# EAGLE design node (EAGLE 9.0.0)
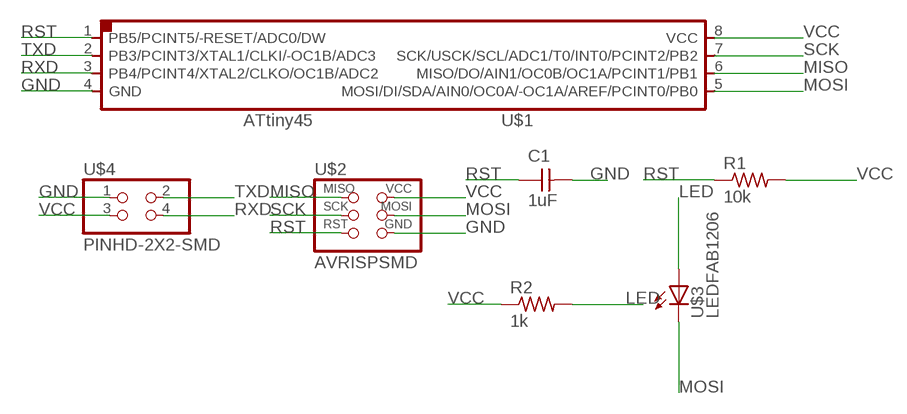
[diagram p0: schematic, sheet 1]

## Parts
C1  1uF  CAP-UNPOLARIZEDFAB  [C1206FAB]
R1  10k  RES-US1206FAB  [R1206FAB]
R2  1k  RES-US1206FAB  [R1206FAB]
U$1  ATTINY45SI  [SOIC8]
U$2  AVRISPSMD  [2X03SMD]
U$3  LEDFAB1206  [LED1206FAB]
U$4  PINHD-2X2-SMD  [2X02SMD]

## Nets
GND: C1.2 U$1.4(GND) U$2.6(GND) U$4.1
LED: R2.2 U$3.1(A)
MISO: U$1.6(MISO/DO/AIN1/OC0B/OC1A/PCINT1/PB1) U$2.1(MISO)
MOSI: U$1.5(MOSI/DI/SDA/AIN0/OC0A/-OC1A/AREF/PCINT0/PB0) U$2.4(MOSI) U$3.2(C)
RST: C1.1 R1.1 U$1.1(PB5/PCINT5/-RESET/ADC0/DW) U$2.5(RST)
RXD: U$1.3(PB4/PCINT4/XTAL2/CLKO/OC1B/ADC2) U$4.4
SCK: U$1.7(SCK/USCK/SCL/ADC1/T0/INT0/PCINT2/PB2) U$2.3(SCK)
TXD: U$1.2(PB3/PCINT3/XTAL1/CLKI/-OC1B/ADC3) U$4.2
VCC: R1.2 R2.1 U$1.8(VCC) U$2.2(VCC) U$4.3

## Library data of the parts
C1 = fab:CAP-UNPOLARIZED
R1 R2 = fab:RES-US: Resistor (US Symbol)
U$1 = fab:ATTINY45
U$2 = fab:AVRISP
U$3 = fab:LED: LED
U$4 = fab:PINHD-2X2-SMD

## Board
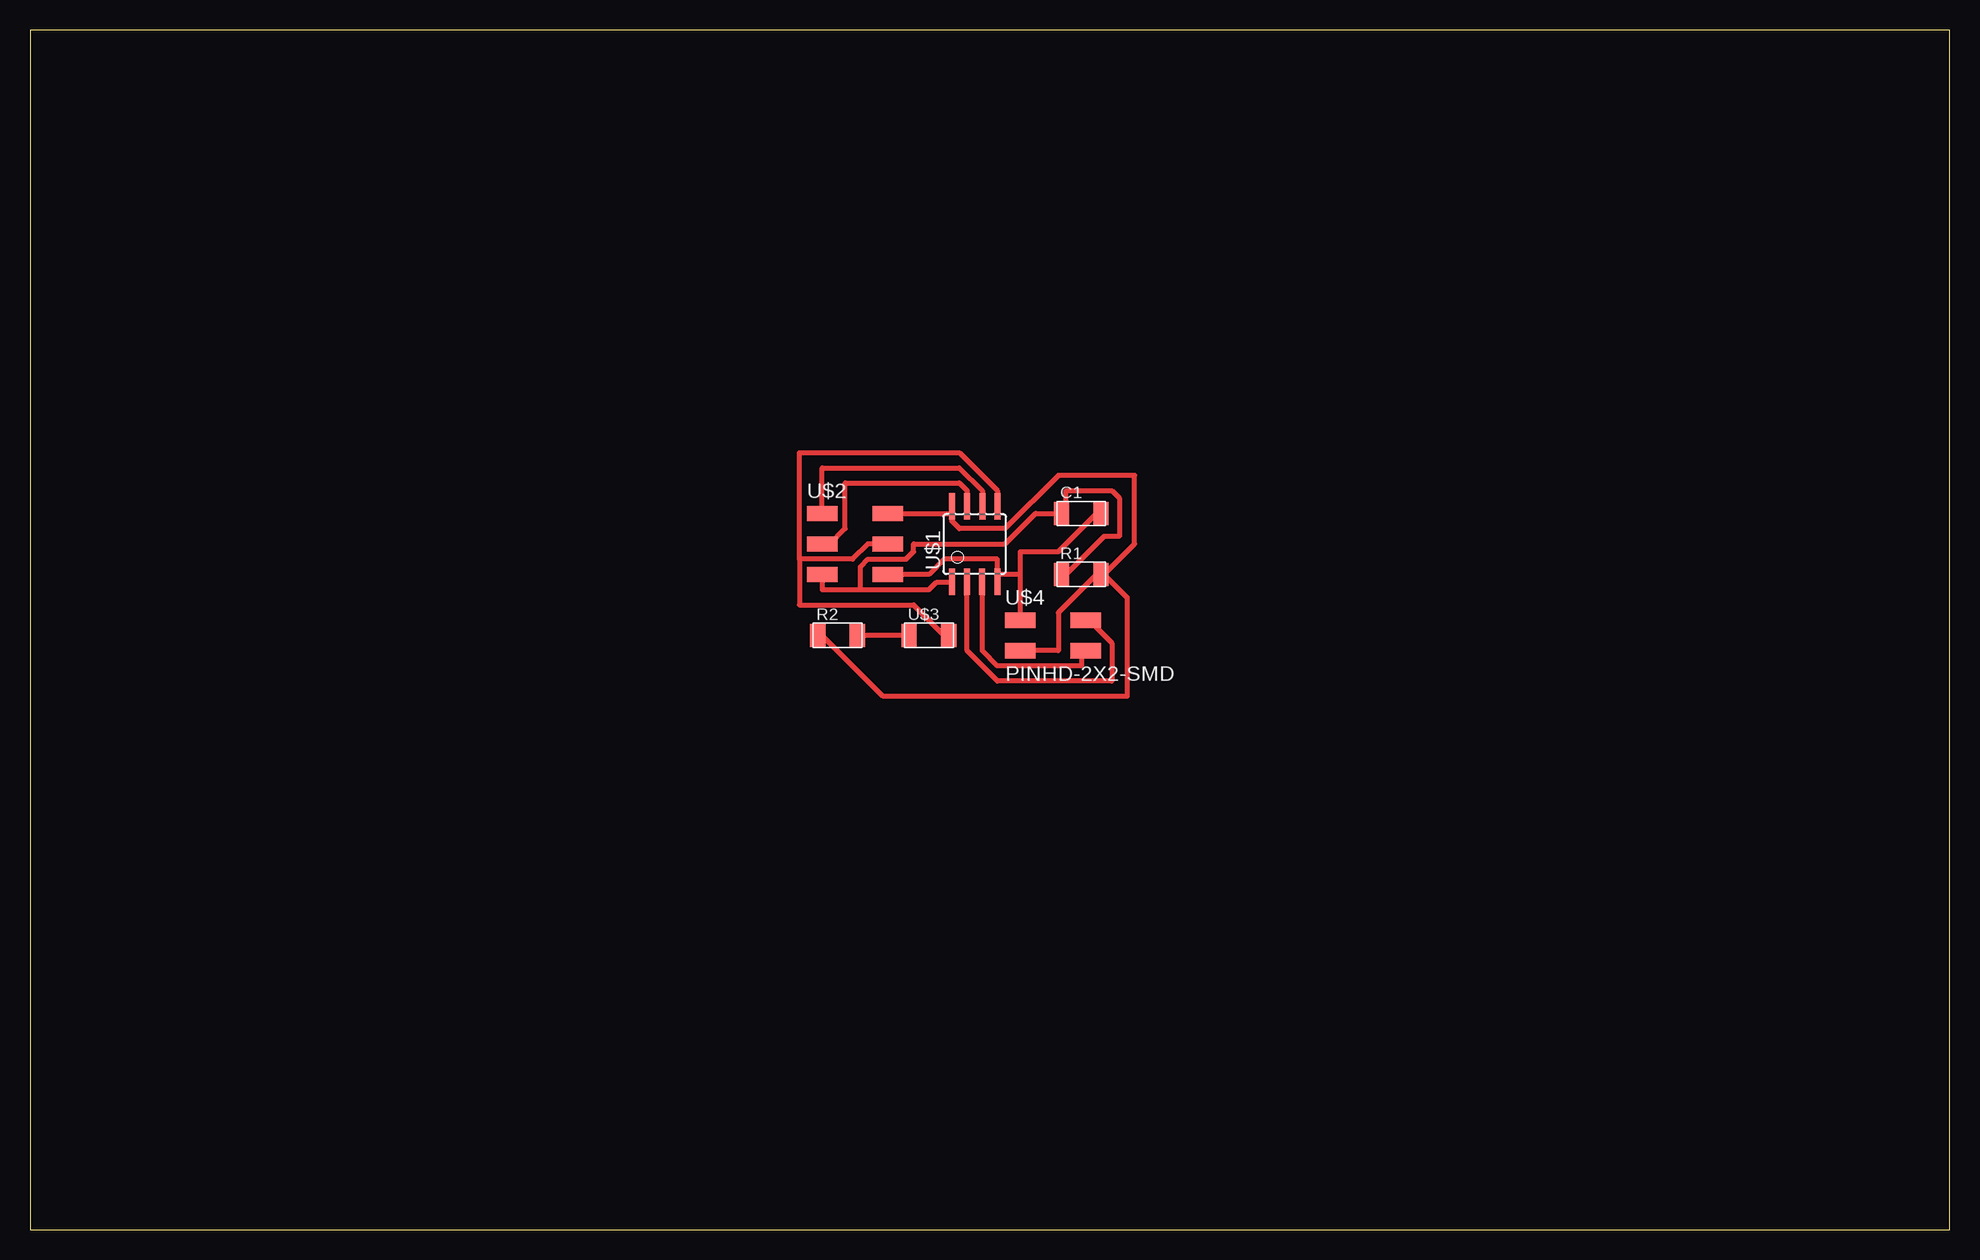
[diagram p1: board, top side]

Size 160 x 100 mm. Coordinates in mm from the lower left corner, seen from the top.
Outline: 0,0 160,0 160,100 0,100 0,0
Copper layers (1*16): Top 0.035mm / dielectric 1.5mm / Bottom 0.035mm
Design rules "default *": minimum track width 16mil, minimum drill 0.35mm, track to track 16mil, track to pad 16mil, pad to pad 16mil, via to via 16mil, smd to smd 16mil, copper to edge 40mil, drill to drill 6mil, minimum pad ring 10mil, minimum via ring 8mil, stop-mask expansion 4mil, vias tented up to drill 0mil, thermal gap 10mil

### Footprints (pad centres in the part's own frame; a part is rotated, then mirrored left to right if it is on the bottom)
C1206FAB = smd 1.27 x 1.905: 1 -1.651,0; 2 1.651,0
R1206FAB = smd 1.27 x 1.905: 1 -1.651,0; 2 1.651,0
SOIC8 = smd 0.5 x 2.2: 1 -1.905,-3.154; 2 -0.645,-3.154; 3 0.625,-3.154; 4 1.895,-3.154; 5 1.905,3.154; 6 0.635,3.154; 7 -0.635,3.154; 8 -1.905,3.154
2X03SMD = smd 2.54 x 1.27: 1 -2.54,2.54; 2 2.92,2.54; 3 -2.54,0; 4 2.92,0; 5 -2.54,-2.54; 6 2.92,-2.54
LED1206FAB = smd 1.27 x 1.905: 1 -1.651,0; 2 1.651,0
2X02SMD = smd 2.54 x 1.27: 1 -2.54,1.27; 2 2.92,1.27; 3 -2.54,-1.27; 4 2.92,-1.27

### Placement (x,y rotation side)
C1  87.63,59.69 0 top
R1  87.63,54.61 0 top
R2  67.31,49.53 0 top
U$1  78.74,57.15 0 top
U$2  68.58,57.15 0 top
U$3  74.93,49.53 0 top
U$4  85.09,49.53 0 top

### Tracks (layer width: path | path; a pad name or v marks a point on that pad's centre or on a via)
GND
  Top 0.406: U$4.1 82.55,54.61 | 82.55,54.61 82.55,56.52 85.72,56.52 88.9,59.69 C1.2 | 82.55,54.61 80.64,54.61 | U$2.6 74.93,54.61 76.2,55.88 80.64,55.88 80.64,54.61 | 80.64,54.61 U$1.4
LED
  Top 0.406: U$3.1 R2.2
MISO
  Top 0.406: U$1.6 79.38,61.59 77.47,63.5 66.04,63.5 U$2.1
MOSI
  Top 0.406: 64.14,55.88 64.14,52.07 73.66,52.07 76.2,49.53 U$3.2 | 64.14,55.88 68.58,55.88 69.85,57.15 U$2.4 | U$1.5 80.64,61.59 77.47,64.77 64.14,64.77 64.14,55.88
RST
  Top 0.406: R1.1 86.36,54.61 89.53,57.78 90.81,57.78 90.81,60.96 90.17,61.59 86.36,61.59 86.36,59.69 C1.1 83.82,59.69 81.28,57.15 73.66,57.15 73.66,56.52 73.03,55.88 69.85,55.88 69.22,55.24 69.22,53.34 | 69.22,53.34 66.04,53.34 U$2.5 | 69.22,53.34 74.93,53.34 75.56,53.98 76.83,53.98 U$1.1
RXD
  Top 0.406: U$1.3 79.38,53.98 79.38,48.26 80.64,46.99 87.63,46.99 87.63,48.26 U$4.4
SCK
  Top 0.406: U$1.7 78.11,61.59 77.47,62.23 67.94,62.23 67.94,58.42 66.67,57.15 U$2.3
TXD
  Top 0.406: U$1.2 78.11,53.98 78.11,48.26 80.64,45.72 90.17,45.72 90.17,48.9 88.27,50.8 U$4.2
VCC
  Top 0.406: U$2.2 76.83,59.69 | 89.53,54.61 91.44,52.7 91.44,44.45 71.12,44.45 66.04,49.53 R2.1 | U$4.3 85.72,48.26 85.72,51.44 88.9,54.61 R1.2 89.53,54.61 | 76.83,59.69 76.83,59.05 77.47,58.42 81.28,58.42 85.72,62.87 92.08,62.87 92.08,57.15 89.53,54.61 | 76.83,59.69 U$1.8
